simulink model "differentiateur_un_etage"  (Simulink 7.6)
settings: Solver=ode15s  StartTime=0.0  StopTime=1  RelTol=1e-3
StopFcn:
  | close all, clc
  | load v2_v1.mat
  | plot(x(1,:),x(2,:),x(1,:),x(3,:),x(1,:),x(4,:))
  | axis([0 1 -2 1.5])
  | title('Montage différentiateur')
  | xlabel('temps')
  | grid
undefined symbols (not defined in the file or in its folder): sigbuilder_block
libraries: fl_lib x14, nesl_utility x4

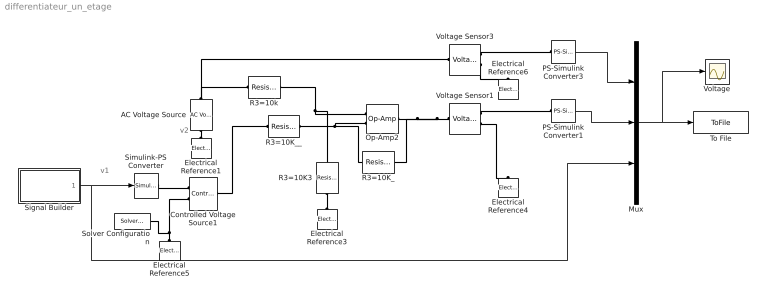
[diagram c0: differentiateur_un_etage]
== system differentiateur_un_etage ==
  note: v2
  note: v1
  AC Voltage Source : fl_lib/Electrical/Electrical Sources/AC Voltage Source  DialogController=NetworkEngine.DynNeDlgSource  SystemSampleTime=-1  amp=1 V  shift=0 rad  omega=1 Hz  i_Log=off  v_Log=off  LocalVarNames=|current|voltage|power  LocalVarDescs=|Current (A)|Voltage (V)|Power (W)  LocalVarLogging=[0 0 0]
  Controlled Voltage Source1 : fl_lib/Electrical/Electrical Sources/Controlled Voltage Source  DialogController=NetworkEngine.DynNeDlgSource  SystemSampleTime=-1  i_Log=off  v_Log=off  LocalVarNames=|current|voltage|power  LocalVarDescs=|Current (A)|Voltage (V)|Power (W)  LocalVarLogging=[0 0 0]
  Electrical Reference{1,3..6} (5 alike) : fl_lib/Electrical/Electrical Elements/Electrical Reference  DialogController=NetworkEngine.DynNeDlgSource  SystemSampleTime=-1  i_Log=off  LocalVarNames=|i  LocalVarDescs=|i  LocalVarLogging=[]
  Mux : Mux  Inputs=3
  Op-Amp2 : fl_lib/Electrical/Electrical Elements/Op-Amp  DialogController=NetworkEngine.DynNeDlgSource  SystemSampleTime=-1  i1_Log=off  v1_Log=off  outI_Log=off  LocalVarNames=|i1|v1|outI  LocalVarDescs=|i1|v1|outI  LocalVarLogging=[]
  PS-Simulink Converter1 : nesl_utility/PS-Simulink Converter  DialogController=NetworkEngine.DynNeUtilDlgSource  SystemSampleTime=-1  PhysicalDomain=network_engine_domain  LeftPortType=input  RightPortType=output  SubClassName=ps_output  Unit=1  AffineConversion=off
  PS-Simulink Converter3 : nesl_utility/PS-Simulink Converter  DialogController=NetworkEngine.DynNeUtilDlgSource  SystemSampleTime=-1  PhysicalDomain=network_engine_domain  LeftPortType=input  RightPortType=output  SubClassName=ps_output  Unit=1  AffineConversion=off
  R3=10K3 : fl_lib/Electrical/Electrical Elements/Resistor  DialogController=NetworkEngine.DynNeDlgSource  SystemSampleTime=-1  R=10e3 Ohm  i_Log=off  v_Log=off  LocalVarNames=|current|voltage|power  LocalVarDescs=|Resistor current (A)|Voltage across resistor (V)|Power (W)  LocalVarLogging=[0 0 0]
  R3=10K_ : fl_lib/Electrical/Electrical Elements/Resistor  DialogController=NetworkEngine.DynNeDlgSource  SystemSampleTime=-1  R=10e3 Ohm  i_Log=off  v_Log=off  LocalVarNames=|current|voltage|power  LocalVarDescs=|Resistor current (A)|Voltage across resistor (V)|Power (W)  LocalVarLogging=[0 0 0]
  R3=10K__ : fl_lib/Electrical/Electrical Elements/Resistor  DialogController=NetworkEngine.DynNeDlgSource  SystemSampleTime=-1  R=10e3 Ohm  i_Log=off  v_Log=off  LocalVarNames=|current|voltage|power  LocalVarDescs=|Resistor current (A)|Voltage across resistor (V)|Power (W)  LocalVarLogging=[0 0 0]
  R3=10k : fl_lib/Electrical/Electrical Elements/Resistor  DialogController=NetworkEngine.DynNeDlgSource  SystemSampleTime=-1  R=10e3 Ohm  i_Log=off  v_Log=off  LocalVarNames=|current|voltage|power  LocalVarDescs=|Resistor current (A)|Voltage across resistor (V)|Power (W)  LocalVarLogging=[0 0 0]
  Signal Builder : Subsystem  Tag=STV Subsys  LoadFcn=sigbuilder_block('load');  StartFcn=sigbuilder_block('start');  StopFcn=sigbuilder_block('stop');  ClipboardFcn=sigbuilder_block('clipboard');
  Simulink-PS Converter : nesl_utility/Simulink-PS Converter  DialogController=NetworkEngine.DynNeUtilDlgSource  SystemSampleTime=-1  PhysicalDomain=network_engine_domain  LeftPortType=input  RightPortType=output  SubClassName=ps_input  Unit=1  AffineConversion=off  InputFilterTimeConstant=.001  UdotUserProvided=0
  Solver Configuration : nesl_utility/Solver Configuration  DialogController=NetworkEngine.DynNeUtilDlgSource  SystemSampleTime=-1  PhysicalDomain=network_engine_domain  LeftPortType=input  RightPortType=generic  SubClassName=solver  Accelerate=off  Profile=off  ResidualTolerance=1e-9  MaxNonlinIter=12  MaxModeIter=2  DoFixedCost=off  UseLocalSampling=off  DoDC=off  LinearAlgebra=Sparse  LocalSolverSampleTime=.001  LocalSolverChoice=NE_BACKWARD_EULER_ADVANCER  UseLocalSolver=off
  To File : ToFile  Filename=v2_v1  MatrixName=x
  Voltage : Scope
  Voltage Sensor1 : fl_lib/Electrical/Electrical Sensors/Voltage Sensor  DialogController=NetworkEngine.DynNeDlgSource  SystemSampleTime=-1  i1_Log=off  v1_Log=off  LocalVarNames=|i1|v1  LocalVarDescs=|i1|v1  LocalVarLogging=[]
  Voltage Sensor3 : fl_lib/Electrical/Electrical Sensors/Voltage Sensor  DialogController=NetworkEngine.DynNeDlgSource  SystemSampleTime=-1  i1_Log=off  v1_Log=off  LocalVarNames=|i1|v1  LocalVarDescs=|i1|v1  LocalVarLogging=[]
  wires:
  Signal Builder/1(Signal 2) -> Simulink-PS Converter/1, Mux/3
  PS-Simulink Converter3/1 -> Mux/1
  Mux/1 -> To File/1, Voltage/1
  PS-Simulink Converter1/1 -> Mux/2
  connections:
  R3=10K__/RConn1 -- R3=10K_/LConn1 -- Op-Amp2/LConn2
  Voltage Sensor1/LConn1 -- R3=10K_/RConn1 -- Op-Amp2/RConn1
  R3=10k/RConn1 -- R3=10K3/LConn1 -- Op-Amp2/LConn1
  R3=10K3/RConn1 -- Electrical Reference3/LConn1
  Voltage Sensor1/RConn2 -- Electrical Reference4/LConn1
  Voltage Sensor1/RConn1 -- PS-Simulink Converter1/LConn1
  AC Voltage Source/LConn1 -- R3=10k/LConn1 -- Voltage Sensor3/LConn1
  AC Voltage Source/RConn1 -- Electrical Reference1/LConn1
  Controlled Voltage Source1/LConn1 -- R3=10K__/LConn1
  Simulink-PS Converter/RConn1 -- Controlled Voltage Source1/RConn1
  Electrical Reference5/LConn1 -- Controlled Voltage Source1/RConn2 -- Solver Configuration/RConn1
  Voltage Sensor3/RConn1 -- PS-Simulink Converter3/LConn1
  Voltage Sensor3/RConn2 -- Electrical Reference6/LConn1

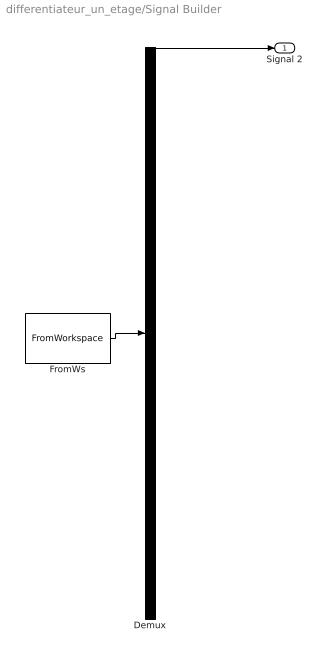
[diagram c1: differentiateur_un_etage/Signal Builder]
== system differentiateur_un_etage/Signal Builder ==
  Demux : Demux  Tag=STV Demux  Outputs=1
  FromWs : FromWorkspace  Tag=STV FromWs  VariableName=tuvar  SampleTime=0  SigBuilderData=DataTag0  VnvData=DataTag1
  Signal 2 : Outport  Tag=STV Outport
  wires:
  Demux/1 -> Signal 2/1
  FromWs/1 -> Demux/1
